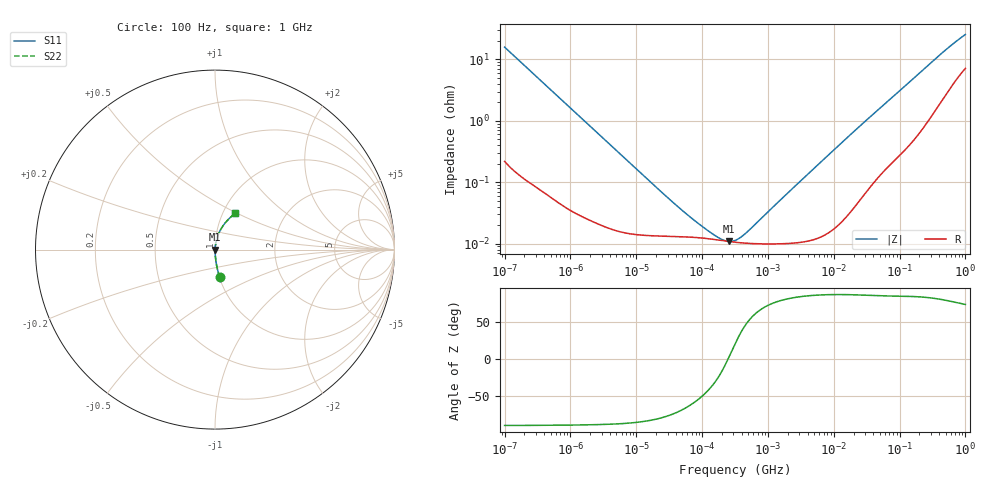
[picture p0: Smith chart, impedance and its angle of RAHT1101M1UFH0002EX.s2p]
! RAHT1101M1UFH0002EX  S-PARAMETER MODEL  (AEC-Q200 qualified)
! Model Generated by ELNA Corporation (http://www.ty-top.com)
! Version 1.0
! ELNA Control No. 201214
! Copyright (c) 2020 ELNA CO.,LTD. All Rights Reserved.
! Products Name : CONDUCTIVE POLYMER HYBRID ALUMINUM ELECTROLYTIC CAPACITORS
! Characteristics :
!  Capacitance  :  100uF  ,  Rated voltage  :  50V
!  Operating Temp. Range  :  -55 to +105 degC  ,  Endurance  :  10000hr at 105 degC
!  Dimension D  :  10mm  ,  Dimension L  :  10mm
! Frequency Range : 100Hz - 1GHz
! External Node Assignments :
!  1  o---| |---o  2
# MHz S RI R 50
!Freq[MHz].  S11 Real  S11 Imag  S21 Real  S21 Imag  S12 Real  S12 Imag  S22 Real  S22 Imag
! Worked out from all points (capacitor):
!   401 points, 100 Hz to 1 GHz, reference 50 ohm
!   read as one part in series: C = 100 uF near 108 Hz
!   lowest |Z| = 10.8 mohm at 258.5 kHz (marker M1)
!   series resonance near 247.3 kHz, so ESL is about 4.1 nH
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0.0001  0.0266 -0.1542  0.9734 0.1542  0.9734 0.1542  0.0266 -0.1542
0.000113  0.0212 -0.1375  0.9788 0.1375  0.9788 0.1375  0.0212 -0.1375
0.000183  0.00868 -0.0861  0.9913 0.0861  0.9913 0.0861  0.00868 -0.0861
0.000309  0.00347 -0.0515  0.9965 0.0515  0.9965 0.0515  0.00347 -0.0515
0.000613  0.00117 -0.0262  0.9988 0.0262  0.9988 0.0262  0.00117 -0.0262
0.001488  0.000394 -0.0109  0.9996 0.0109  0.9996 0.0109  0.000394 -0.0109
0.022131  0.000133 -0.00074  0.9999 0.00074  0.9999 0.00074  0.000133 -0.00074
0.053703  0.000129 -0.000298  0.9999 0.000298  0.9999 0.000298  0.000129 -0.000298
0.110917  0.000122 -0.000127  0.9999 0.000127  0.9999 0.000127  0.000122 -0.000127
0.187284  0.000113 -4.23e-05  0.9999 4.23e-05  0.9999 4.23e-05  0.000113 -4.23e-05
0.220039  0.00011 -1.79e-05  0.9999 1.79e-05  0.9999 1.79e-05  0.00011 -1.79e-05
0.258523  0.000108 6.9e-06  0.9999 -6.9e-06  0.9999 -6.9e-06  0.000108 6.9e-06
0.316228  0.000105 3.92e-05  0.9999 -3.92e-05  0.9999 -3.92e-05  0.000105 3.92e-05
0.386812  0.000103 7.4e-05  0.9999 -7.4e-05  0.9999 -7.4e-05  0.000103 7.4e-05
0.492606  0.000101 0.000121  0.9999 -0.000121  0.9999 -0.000121  0.000101 0.000121
4.704354  0.000116 0.00157  0.9999 -0.00157  0.9999 -0.00157  0.000116 0.00157
21.75204  0.000471 0.00717  0.9995 -0.00717  0.9995 -0.00717  0.000471 0.00717
69.9842  0.00234 0.0217  0.9977 -0.0217  0.9977 -0.0217  0.00234 0.0217
184.0772  0.00855 0.0542  0.9915 -0.0542  0.9915 -0.0542  0.00855 0.0542
429.0422  0.034 0.1157  0.966 -0.1157  0.966 -0.1157  0.034 0.1157
695.825  0.0713 0.165  0.9287 -0.165  0.9287 -0.165  0.0713 0.165
1000  0.113 0.2026  0.887 -0.2026  0.887 -0.2026  0.113 0.2026
